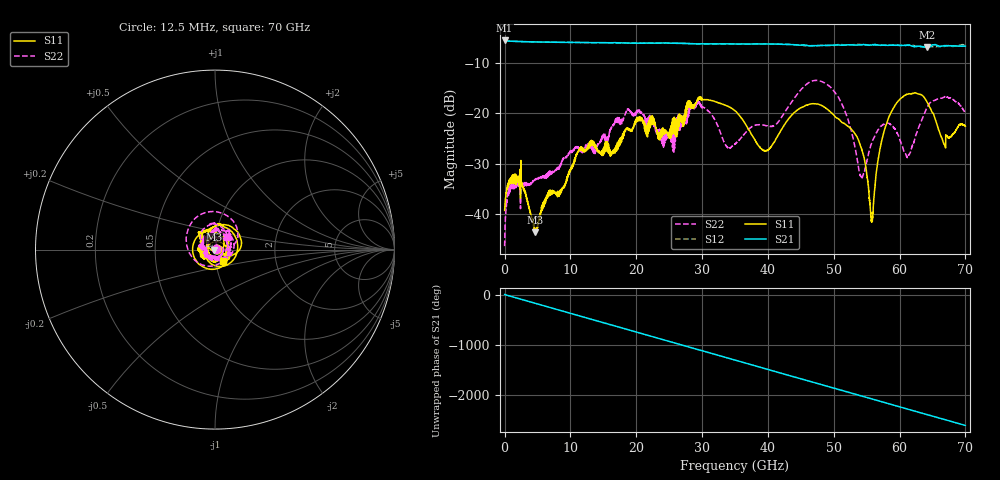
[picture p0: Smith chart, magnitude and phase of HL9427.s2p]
! 5/9/2023 1:24:54 PM
! H:\PROTOTYPE_DATA\110GHZ-ATTN\A2.S2P
! CHANNEL.1
! TR.MEASUREMENT
! CORRECTED.DATA
! RF.CORRECTION: FULL.TWO.PORT.CAL.PORT.1.2
! AVERAGING: 1 PointByPoint
! IF.BANDWIDTH: 1KHZ
! SWEEPTYPE:  FREQ.SWEEP(Linear)
! Reference Plane Port Info
! PORT:  PORT1  PORT2
! DISTANCE:  0  m  0  m
! TIME:  0  s  0  s
! PHASE.OFFSET:  0 °  0 °
! LOSS:  0  dB  0  dB
! REF.LOSS:  0  dB  0  dB
! REF.FREQ:  0  Hz  0  Hz
! Power Info
! POWER:  -10  dBm  -10  dBm
! EFF.POWER:  -10  dBm  -10  dBm
! POWER(>54G):  -10  dBm  -10  dBm
! EFF.POWER(>54G):  -10  dBm  -10  dBm
! SOURCE.ATTEN:  0  dB  0  dB
! TEST.ATTEN:  0  dB  0  dB
# GHZ S RI R 50.0
! FREQ.GHZ  S11RE  S11IM  S21RE  S21IM  S12RE  S12IM  S22RE  S22IM
!; PortSelection: Port_12
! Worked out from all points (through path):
!   5600 points, 12.5 MHz to 70 GHz, reference 50 ohm
!   highest |S21| = -5.46 dB at 12.5 MHz (marker M1); lowest = -6.9 dB at 64.14 GHz (marker M2)
!   group delay of S21, straight-line fit = 104 ps
!   lowest |S11| = -43.7 dB at 4.625 GHz (marker M3), VSWR 1.01, Z = 49.4 + j0.0186 ohm
!   |S11| at or under -10 dB: start of sweep to end of sweep
!   |S22| runs from -46.5 to -13.4 dB; largest |S21 - S12| = 0.033
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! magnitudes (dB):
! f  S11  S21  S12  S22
! 12.5 MHz  -39.4  -5.5  -5.5  -46.5
! 750 MHz  -33.2  -5.6  -5.6  -34.5
! 2.237 GHz  -33.6  -5.7  -5.7  -34.0
! 4.625 GHz  -43.7  -5.8  -5.7  -33.3
! 11.69 GHz  -26.7  -5.9  -5.9  -27.6
! 16.39 GHz  -27.6  -5.9  -5.9  -22.7
! 18.75 GHz  -23.0  -6.0  -6.0  -19.1
! 23.35 GHz  -24.3  -6.0  -6.0  -23.5
! 29.5 GHz  -17.0  -6.1  -6.1  -17.7
! 35.01 GHz  -19.5  -6.2  -6.2  -26.1
! 39.66 GHz  -27.4  -6.2  -6.1  -22.4
! 46.67 GHz  -18.1  -6.5  -6.5  -13.6
! 50.69 GHz  -21.1  -6.4  -6.3  -16.7
! 53.46 GHz  -24.5  -6.4  -6.3  -28.3
! 54.34 GHz  -27.5  -6.3  -6.4  -32.8
! 55.75 GHz  -41.3  -6.4  -6.4  -26.0
! 56.98 GHz  -27.5  -6.4  -6.4  -22.8
! 58.34 GHz  -20.9  -6.4  -6.4  -22.0
! 61.3 GHz  -16.1  -6.4  -6.3  -28.5
! 64.14 GHz  -17.6  -6.9  -6.7  -18.9
! 66.65 GHz  -25.9  -6.5  -6.6  -16.8
! 70 GHz  -22.6  -6.6  -6.4  -20.0
